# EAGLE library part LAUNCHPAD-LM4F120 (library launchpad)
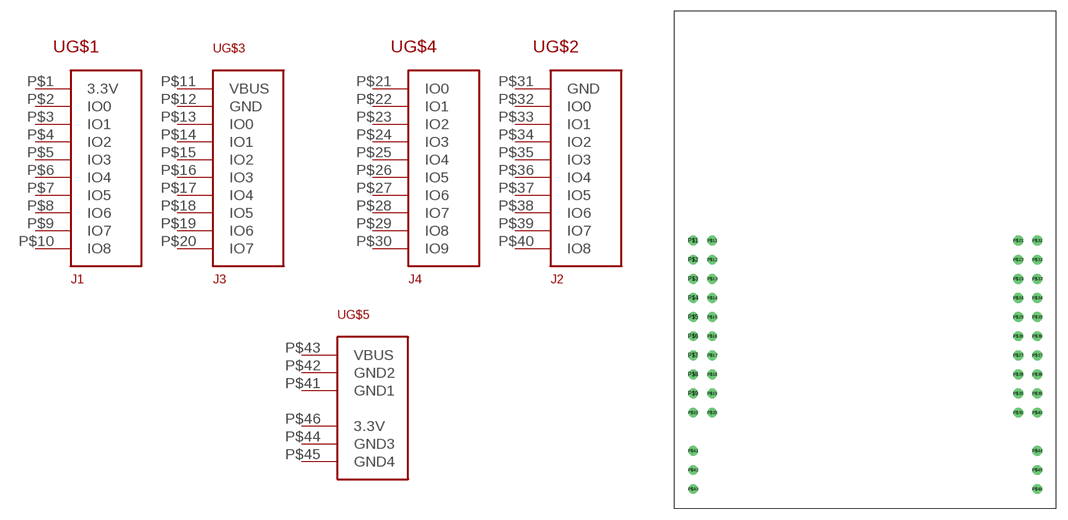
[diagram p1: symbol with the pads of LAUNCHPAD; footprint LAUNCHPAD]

Designator prefix -; gates G$1=LAUNCHPAD-J1 G$2=LAUNCHPAD-J2 G$3=LAUNCHPAD-J3 G$4=LAUNCHPAD-J4 G$5=LAUNCHPAD-HD

## LAUNCHPAD-LM4F120  [LAUNCHPAD]
P$1  G$1:3.3V
P$2  G$1:IO0
P$3  G$1:IO1
P$4  G$1:IO2
P$5  G$1:IO3
P$6  G$1:IO4
P$7  G$1:IO5
P$8  G$1:IO6
P$9  G$1:IO7
P$10  G$1:IO8
P$11  G$3:VBUS
P$12  G$3:GND
P$13  G$3:IO0
P$14  G$3:IO1
P$15  G$3:IO2
P$16  G$3:IO3
P$17  G$3:IO4
P$18  G$3:IO5
P$19  G$3:IO6
P$20  G$3:IO7
P$21  G$4:IO0
P$22  G$4:IO1
P$23  G$4:IO2
P$24  G$4:IO3
P$25  G$4:IO4
P$26  G$4:IO5
P$27  G$4:IO6
P$28  G$4:IO7
P$29  G$4:IO8
P$30  G$4:IO9
P$31  G$2:GND
P$32  G$2:IO0
P$33  G$2:IO1
P$34  G$2:IO2
P$35  G$2:IO3
P$36  G$2:IO4
P$37  G$2:IO5
P$38  G$2:IO6
P$39  G$2:IO7
P$40  G$2:IO8
P$41  G$5:GND1
P$42  G$5:GND2
P$43  G$5:VBUS
P$44  G$5:GND3
P$45  G$5:GND4
P$46  G$5:3.3V

## Footprint LAUNCHPAD (pad centres in mm)
drill 0.8: P$1 0,0; P$2 0,-2.54; P$3 0,-5.08; P$4 0,-7.62; P$5 0,-10.16; P$6 0,-12.7; P$7 0,-15.24; P$8 0,-17.78; P$9 0,-20.32; P$10 0,-22.86; P$11 2.54,0; P$12 2.54,-2.54; P$13 2.54,-5.08; P$14 2.54,-7.62; P$15 2.54,-10.16; P$16 2.54,-12.7; P$17 2.54,-15.24; P$18 2.54,-17.78; P$19 2.54,-20.32; P$20 2.54,-22.86; P$21 43.18,0; P$22 43.18,-2.54; P$23 43.18,-5.08; P$24 43.18,-7.62; P$25 43.18,-10.16; P$26 43.18,-12.7; P$27 43.18,-15.24; P$28 43.18,-17.78; P$29 43.18,-20.32; P$30 43.18,-22.86; P$31 45.72,0; P$32 45.72,-2.54; P$33 45.72,-5.08; P$34 45.72,-7.62; P$35 45.72,-10.16; P$36 45.72,-12.7; P$37 45.72,-15.24; P$38 45.72,-17.78; P$39 45.72,-20.32; P$40 45.72,-22.86; P$41 0,-27.94; P$42 0,-30.48; P$43 0,-33.02; P$44 45.72,-27.94; P$45 45.72,-30.48; P$46 45.72,-33.02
